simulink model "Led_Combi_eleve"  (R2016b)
settings: Solver=VariableStepAuto  StartTime=0.0  StopTime=inf  RelTol=1e-3
libraries: realtime_pacer_lib x1

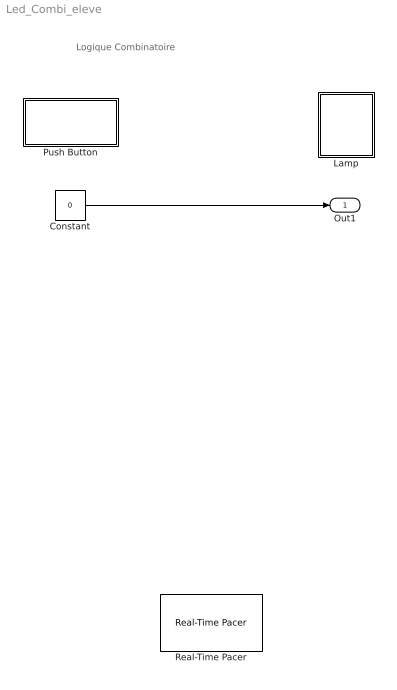
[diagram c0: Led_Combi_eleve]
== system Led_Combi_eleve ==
  note: Logique Combinatoire
  Constant : Constant  Value=0
  Lamp : Subsystem  DialogController=hmiCreateDDGDialog  IsWebBlock=on
  Push Button : Subsystem  DialogController=hmiCreateDDGDialog  IsWebBlock=on
  Real-Time Pacer : realtime_pacer_lib/Real-Time Pacer  simTimePerRealTime=1
  Out1 : Outport
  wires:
  Constant/1 -> Out1/1

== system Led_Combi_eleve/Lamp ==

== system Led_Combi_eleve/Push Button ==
